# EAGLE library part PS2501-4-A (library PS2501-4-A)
Transistor Output Optocouplers Optocoupler 16-pin DIP Source: Datasheet
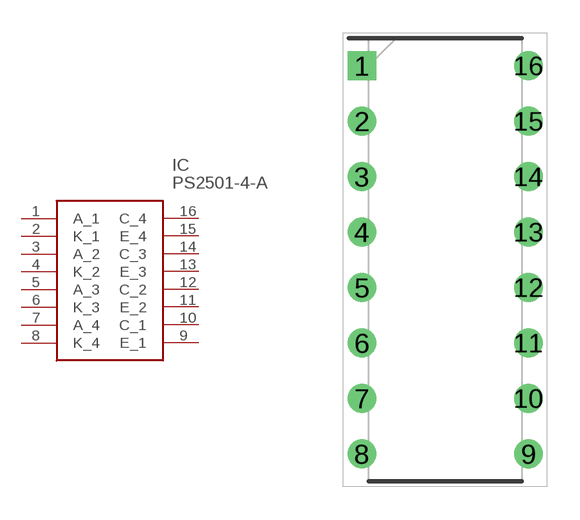
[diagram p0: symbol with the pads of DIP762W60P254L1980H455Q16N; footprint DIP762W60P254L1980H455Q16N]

Designator prefix IC

## PS2501-4-A (Arrow_Part_Number: PS2501-4-A; Arrow_Price-Stock: https://www.arrow.com/en/products/ps2501-4-a/renesas-electronics; Description: Transistor Output Optocouplers Optocoupler 16-pin DIP; Height: 4.55mm; Manufacturer_Name: Renesas Electronics; Manufacturer_Part_Number: PS2501-4-A; Mouser_Part_Number: 551-PS2501-4-A; Mouser_Price-Stock: https://www.mouser.co.uk/ProductDetail/Renesas-Electronics/PS2501-4-A?qs=qSfuJ%252Bfl%2Fd73DT6GctNDSg%3D%3D)  [DIP762W60P254L1980H455Q16N]
1  A_1
2  K_1
3  A_2
4  K_2
5  A_3
6  K_3
7  A_4
8  K_4
9  E_1
10  C_1
11  E_2
12  C_2
13  E_3
14  C_3
15  E_4
16  C_4

## Footprint DIP762W60P254L1980H455Q16N (pad centres in mm)
PS2501-4
drill 0.8 pad 1.2 square: 1 -3.81,8.89
drill 0.8 pad 1.2: 2 -3.81,6.35; 3 -3.81,3.81; 4 -3.81,1.27; 5 -3.81,-1.27; 6 -3.81,-3.81; 7 -3.81,-6.35; 8 -3.81,-8.89; 9 3.81,-8.89; 10 3.81,-6.35; 11 3.81,-3.81; 12 3.81,-1.27; 13 3.81,1.27; 14 3.81,3.81; 15 3.81,6.35; 16 3.81,8.89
